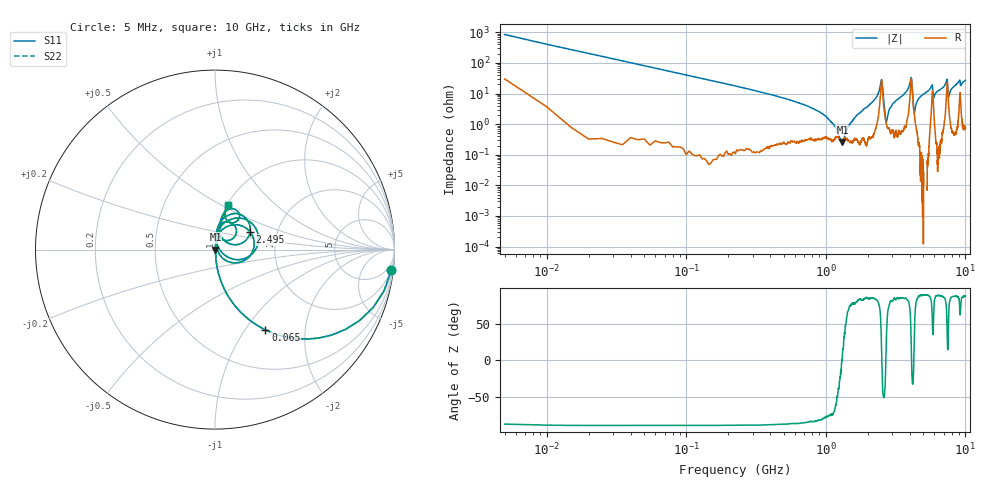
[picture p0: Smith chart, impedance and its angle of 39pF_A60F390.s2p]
! Amotech Co.,Ltd.
! http://www.amotech.co.kr/
! Part Number: A60F390
! These Parameters are Measured in Series Mode Connection
! Operation Temp=25[degC], DC Bias Voltage=0[V]
! Freq. Start=5[MHz] Stop=10[GHz], 2000[Steps]
! Date: Monday, July 20, 2020, 03:40:37
# GHZ S RI R 50.000000
!Freq.(Hz) S11(Real) S11(Imag) S21(Real) S21(Imag) S12(Real) S12(Imag) S22(Real) S22(Imag)
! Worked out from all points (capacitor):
!   2000 points, 5 MHz to 10 GHz, reference 50 ohm
!   read as one part in series: C = 39.1 pF near 55 MHz
!   lowest |Z| = 263 mohm at 1.315 GHz (marker M1)
!   series resonance near 1.304 GHz, so ESL is about 380 pH
!   S11 on the Smith chart (normalised r, x): 5 MHz: 2, -17; 65 MHz: 1.01, -1.25; 2.495 GHz: 1.45, +0.30; 10 GHz: 1.02, +0.54
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0.005  0.9824 -0.1151  0.0176 0.1151  0.0176 0.1151  0.9824 -0.1151
0.065  0.2812 -0.4476  0.7188 0.4476  0.7188 0.4476  0.2812 -0.4476
0.23  0.0301 -0.1668  0.9699 0.1668  0.9699 0.1668  0.0301 -0.1668
0.97  0.00388 -0.0194  0.9961 0.0194  0.9961 0.0194  0.00388 -0.0194
1.315  0.00261 0.000336  0.9974 -0.000336  0.9974 -0.000336  0.00261 0.000336
1.675  0.00349 0.0197  0.9965 -0.0197  0.9965 -0.0197  0.00349 0.0197
2.27  0.0115 0.0674  0.9885 -0.0674  0.9885 -0.0674  0.0115 0.0674
2.495  0.1956 0.099  0.8044 -0.099  0.8044 -0.099  0.1956 0.099
2.715  0.0104 0.00548  0.9896 -0.00548  0.9896 -0.00548  0.0104 0.00548
2.895  0.00659 0.0331  0.9934 -0.0331  0.9934 -0.0331  0.00659 0.0331
3.34  0.0109 0.0677  0.9891 -0.0677  0.9891 -0.0677  0.0109 0.0677
4.075  0.2258 0.121  0.7742 -0.121  0.7742 -0.121  0.2258 0.121
4.31  0.0188 0.0129  0.9812 -0.0129  0.9812 -0.0129  0.0188 0.0129
4.555  0.00733 0.0598  0.9927 -0.0598  0.9927 -0.0598  0.00733 0.0598
5.005  0.00935 0.0947  0.9907 -0.0947  0.9907 -0.0947  0.00935 0.0947
5.755  0.0856 0.1517  0.9144 -0.1517  0.9144 -0.1517  0.0856 0.1517
5.93  0.0297 0.0636  0.9703 -0.0636  0.9703 -0.0636  0.0297 0.0636
6.67  0.0218 0.1361  0.9782 -0.1361  0.9782 -0.1361  0.0218 0.1361
7.365  0.17 0.1768  0.83 -0.1768  0.83 -0.1768  0.17 0.1768
7.575  0.0449 0.0571  0.9551 -0.0571  0.9551 -0.0571  0.0449 0.0571
8.335  0.0349 0.1704  0.9651 -0.1704  0.9651 -0.1704  0.0349 0.1704
10  0.0742 0.2474  0.9258 -0.2474  0.9258 -0.2474  0.0742 0.2474
